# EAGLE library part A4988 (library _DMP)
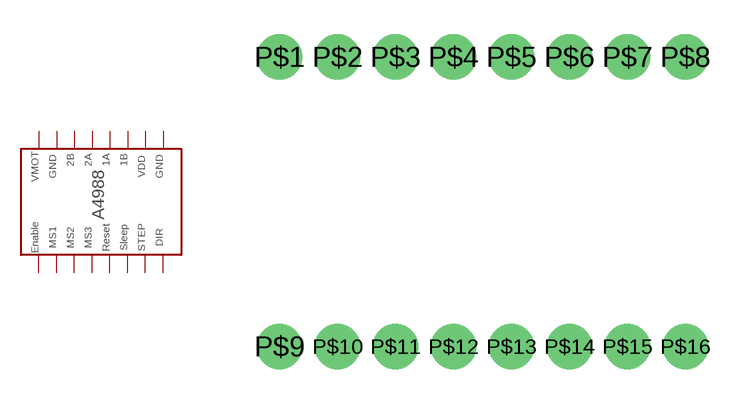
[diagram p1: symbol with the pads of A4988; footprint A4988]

Designator prefix -

## A4988  [A4988]
P$1  VMOT
P$2  GND
P$3  2B
P$4  2A
P$5  1A
P$6  1B
P$7  VDD
P$8  GND2
P$9  ENABLE
P$10  MS1
P$11  MS2
P$12  MS3
P$13  RESET
P$14  SLEEP
P$15  STEP
P$16  DIR

## Footprint A4988 (pad centres in mm)
drill 1.1 pad 2: P$1 0,0; P$2 2.54,0; P$3 5.08,0; P$4 7.62,0; P$5 10.16,0; P$6 12.7,0; P$7 15.24,0; P$8 17.78,0; P$9 0,-12.7; P$10 2.54,-12.7; P$11 5.08,-12.7; P$12 7.62,-12.7; P$13 10.16,-12.7; P$14 12.7,-12.7; P$15 15.24,-12.7; P$16 17.78,-12.7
